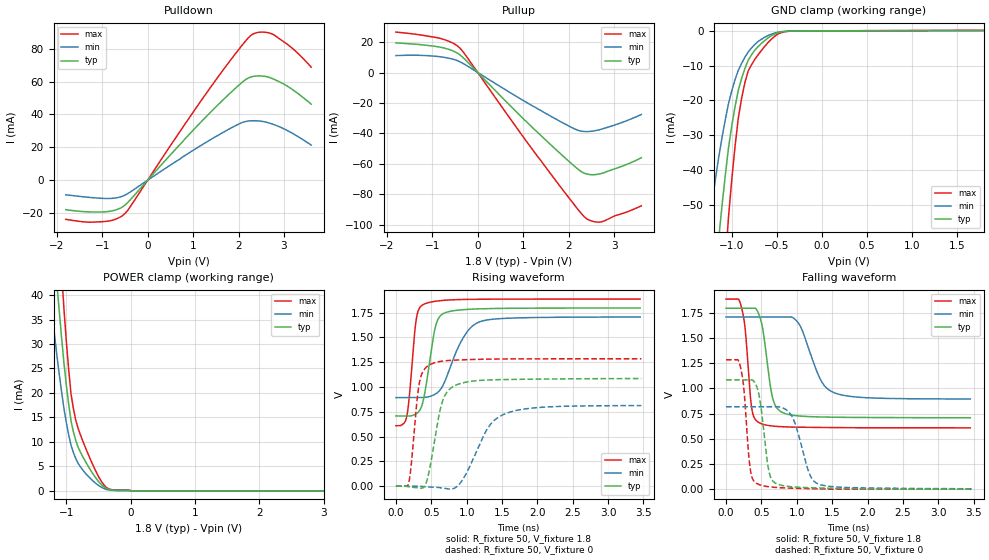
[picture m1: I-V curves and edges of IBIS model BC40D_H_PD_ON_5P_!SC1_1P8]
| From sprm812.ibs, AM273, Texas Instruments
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|   Model Cell BC40D_H_PD_ON_5P_!SC1_1P8
|BC40D_H_PD_ON_5P_!SC1_1P8
[Model]   BC40D_H_PD_ON_5P_!SC1_1P8
Model_type   I/O
Polarity   Non-Inverting
Enable   Active-Low
Vinl =  0.63
Vinh =  1.17
Cref =  15pF
Rref =  100.0000M
Vref =  0V
Vmeas =  0.9
C_comp   2.364487p   2.290698p   2.389419p
|[Input load] weak_pd_on
|[Output drive] fast
|[supplytol] 5
|[temp] ind
[Model Spec]
Vinl   0.63   0.5985   0.6615
Vinh   1.17   1.1115   1.2285
[Temperature Range]   25   125   -40
[Voltage Range]   1.8   1.71   1.89
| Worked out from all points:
|   slope of the pulldown table from 0 to 0.27 V, typ, clamps not added: 32.2 ohm
|   slope of the pullup table from 0 to 0.27 V, typ, clamps not added: 32.5 ohm
|   GND clamp passes 1 mA (typ) near -0.53 V on its own axis
|   POWER clamp passes 1 mA (typ) near -0.43 V on its own axis
|   rising waveform, R_fixture 50, V_fixture 1.8: 20-80 % time 145ps typ, 303ps min, 93.4ps max; typ from 0.708 V to 1.8 V
|   rising waveform, R_fixture 50, V_fixture 0: 20-80 % time 176ps typ, 352ps min, 106ps max; typ from 0 V to 1.09 V
|   falling waveform, R_fixture 50, V_fixture 1.8: 20-80 % time 130ps typ, 266ps min, 88ps max; typ from 1.8 V to 0.709 V
|   falling waveform, R_fixture 50, V_fixture 0: 20-80 % time 113ps typ, 197ps min, 84.3ps max; typ from 1.09 V to 0 V
| Nom Voltages:
|   VDD=1.1, VDDS=1.8, VDDS18=1.8, ESD_BIASFET=0, VSS=0, VSSS=0
| Min Voltages:
|   VDD=1.045, VDDS=1.71, VDDS18=1.71, ESD_BIASFET=0, VSS=0, VSSS=0
| Max Voltages:
|   VDD=1.16, VDDS=1.89, VDDS18=1.89, ESD_BIASFET=0, VSS=0, VSSS=0
[POWER_clamp]
|   voltage   I(typ)   I(min)   I(max)
-1.8V     158.9mA    112.5mA    219.9mA
-1.255V   60.04mA    40.04mA    85.04mA
-1.145V   41.99mA    27.45mA    59.9mA
-1.109V   36.4mA     23.66mA    51.97mA
-1.073V   31.03mA    20.08mA    44.3mA
-1.036V   25.91mA    16.71mA    36.9mA
-927.3mV  14.27mA    9.301mA    19.77mA
-854.5mV  10.33mA    6.623mA    14.48mA
-454.5mV  1.273mA    746.6uA    1.931mA
-309.1mV  221.6uA    137.5uA    298.5uA
18.18mV   0A         0A         0A
3.6V      0A         0A         0A
[Pulldown]
|   voltage   I(typ)   I(min)   I(max)
-1.8V     -17.92mA   -8.85mA    -23.8mA
-1.309V   -19.26mA   -10.37mA   -25.5mA
-927.3mV  -19.22mA   -11.12mA   -25.08mA
-654.5mV  -17.65mA   -10.56mA   -23.13mA
-490.9mV  -14.97mA   -8.985mA   -20.05mA
1.364V    40.78mA    24.32mA    55.69mA
2.073V    59.4mA     35mA       81.9mA
2.291V    62.96mA    36.2mA     88.48mA
2.509V    63.41mA    35.84mA    90.12mA
2.782V    61.38mA    33.82mA    88.42mA
3.218V    54.59mA    28.02mA    79.45mA
3.6V      46.26mA    21.39mA    68.79mA
[Pullup]
|   voltage   I(typ)   I(min)   I(max)
-1.8V     19.47mA    11.11mA    26.55mA
-818.2mV  16.61mA    10.32mA    22.37mA
-545.5mV  14.2mA     8.765mA    19.31mA
-381.8mV  11.35mA    6.927mA    15.71mA
1.255V    -37.58mA   -22.7mA    -52.59mA
2.127V    -61.49mA   -36.97mA   -86.91mA
2.291V    -65.3mA    -38.55mA   -92.97mA
2.4V      -66.65mA   -38.77mA   -96.07mA
2.564V    -67.08mA   -38.3mA    -97.93mA
2.727V    -66.24mA   -37.15mA   -97.99mA
3.273V    -60.4mA    -31.68mA   -91.65mA
3.6V      -55.92mA   -27.55mA   -87.52mA
[GND_clamp]
|   voltage   I(typ)   I(min)   I(max)
-1.8V     -270.2mA   -170.2mA   -430.1mA
-1.255V   -91.66mA   -55.91mA   -148.4mA
-1.145V   -59.91mA   -36.45mA   -97.1mA
-1.109V   -50.48mA   -30.83mA   -81.56mA
-1.073V   -41.73mA   -25.65mA   -67.06mA
-1.036V   -33.67mA   -20.93mA   -53.6mA
-927.3mV  -17.08mA   -11.35mA   -25.06mA
-854.5mV  -10.88mA   -7.624mA   -14.94mA
-781.8mV  -6.944mA   -4.956mA   -9.81mA
-636.4mV  -2.852mA   -1.883mA   -4.567mA
-381.8mV  -107.5uA   -92.09uA   -158.2uA
1.8V      101.9uA    59.12uA    150.8uA
[Ramp]
| variable   typ   min   max
dV/dt_f 0.66466065/0.13257929n 0.49911656/0.27154983n 0.77619839/89.698829p
dV/dt_r 0.66396162/0.17822457n 0.50954501/0.36676031n 0.78038843/0.10690754n
R_load = 50
[Rising Waveform]
R_fixture = 50
V_fixture = 1.8
V_fixture_min = 1.71
V_fixture_max = 1.89
|   time   V(typ)   V(min)   V(max)
0s        708.4mV    893.6mV    610.4mV
151.7ps   708.4mV    893.6mV    698.1mV
187ps     708.4mV    893.6mV    886.2mV
285.7ps   729.7mV    893.6mV    1.675V
390.1ps   875.7mV    895.3mV    1.834V
557.1ps   1.604V     929.2mV    1.866V
690ps     1.748V     1.054V     1.876V
948.8ps   1.78V      1.494V     1.883V
1.197ns   1.789V     1.661V     1.886V
3.453ns   1.798V     1.706V     1.887V
[Rising Waveform]
R_fixture = 50
V_fixture = 0
V_fixture_min = 0
V_fixture_max = 0
|   time   V(typ)   V(min)   V(max)
0s        0V         0V         0V
177.7ps   -5.678mV   0V         25.84mV
328.8ps   -18.25mV   0V         1.031V
407.1ps   0V         -4.568mV   1.183V
481.7ps   192mV      -8.475mV   1.226V
655.2ps   850mV      -18.02mV   1.261V
852.1ps   1.021V     -9.047mV   1.272V
1.295ns   1.071V     580.9mV    1.282V
1.529ns   1.076V     726.2mV    1.283V
3.47ns    1.086V     813.1mV    1.285V
[Falling Waveform]
R_fixture = 50
V_fixture = 1.8
V_fixture_min = 1.71
V_fixture_max = 1.89
|   time   V(typ)   V(min)   V(max)
0s        1.797V     1.71V      1.888V
218.1ps   1.797V     1.71V      1.807V
270.7ps   1.797V     1.71V      1.589V
362ps     1.797V     1.71V      808.3mV
469.7ps   1.727V     1.71V      659.2mV
652.9ps   922.5mV    1.71V      627.3mV
794.5ps   762.4mV    1.71V      619.9mV
1.03ns    727.2mV    1.643V     615.4mV
1.517ns   714.5mV    961.5mV    611.3mV
3.453ns   709.3mV    895.6mV    609.1mV
[Falling Waveform]
R_fixture = 50
V_fixture = 0
V_fixture_min = 0
V_fixture_max = 0
|   time   V(typ)   V(min)   V(max)
0s        1.086V     818.9mV    1.285V
203.8ps   1.086V     818.9mV    1.215V
252.5ps   1.086V     818.9mV    993.6mV
341.7ps   1.086V     818.9mV    202.9mV
444.1ps   996.2mV    818.9mV    52.9mV
601.7ps   194.3mV    818.9mV    24.37mV
713.9ps   54.08mV    818.9mV    16.74mV
935.6ps   23.34mV    719.1mV    9.569mV
1.302ns   11.97mV    51.89mV    2.858mV
3.47ns    0V         3.836mV    0V
